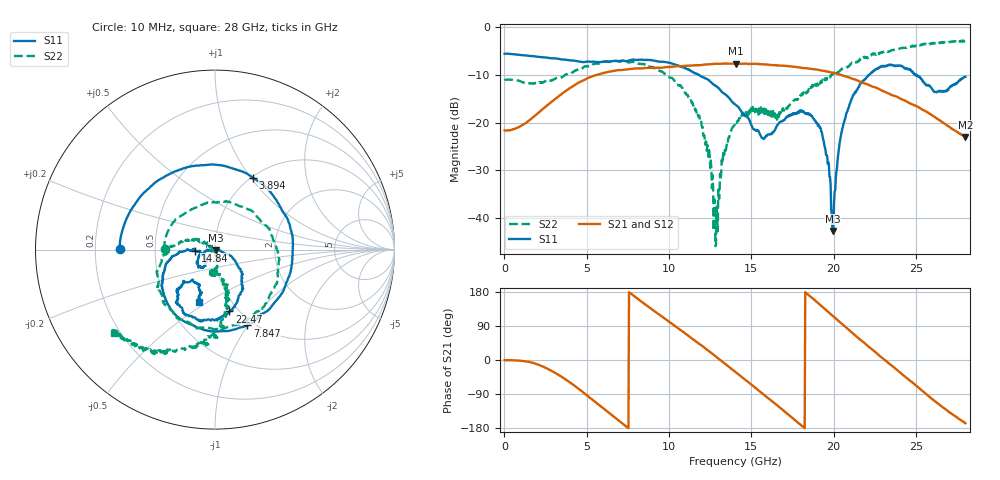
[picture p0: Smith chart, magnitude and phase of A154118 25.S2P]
!  2-Port S-parameters saved by WinCal
! VAR MeasName=S-Parameters (CALIBRATED_DATA) read from VNA (N5230A)
! VAR MeasDate=2015-9-10 14:36:17
! VAR NAME=A154118 25
! VAR FILENAME=A154118 25.S2P
! VAR DATE=2015-9-10 14:36:17
! VAR PHYS_PORTS=1,2
# Hz S DB R 50
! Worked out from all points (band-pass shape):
!   801 points, 10 MHz to 28 GHz, reference 50 ohm
!   highest |S21| = -7.57 dB at 14.07 GHz (marker M1); lowest = -23.0 dB at 28 GHz (marker M2)
!   |S21| within 3 dB of the highest: 5.095 GHz to 20.97 GHz (15.88 GHz wide, 122 % of centre)
!   lowest |S11| = -42.7 dB at 19.95 GHz (marker M3), VSWR 1.01, Z = 50.6 - j0.347 ohm
!   |S11| at or under -10 dB: 11.84 GHz to 22.14 GHz (10.3 GHz wide, 60.6 % of centre); 24.97935 GHz to 25.0482 GHz (68.84 MHz wide, 0.275 % of centre); 25.07 GHz to end of sweep
!   |S22| runs from -45.9 to -2.7 dB; largest |S21 - S12| = 0.0078
!   S11 on the Smith chart (normalised r, x): 10 MHz: 0.31, +0.00; 3.894 GHz: 1.01, +1.02; 7.847 GHz: 0.93, -0.99; 14.84 GHz: 0.80, -0.01; 22.47 GHz: 0.91, -0.71; 28 GHz: 0.71, -0.46
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1e7  -5.53 179.6  -21.62 -0.2  -21.64 0.1  -11.15 179.9
2.10925e9  -6.18 120.3  -17.80 -13.3  -17.80 -13.0  -11.46 96.2
3.893612e9  -6.87 62.3  -12.93 -56.5  -12.89 -56.5  -9.76 16.3
4.698325e9  -7.25 33.6  -11.28 -82.5  -11.26 -82.8  -8.61 -19.1
7.8472e9  -6.76 -66.9  -8.65 169.8  -8.63 169.8  -7.18 -119.2
9.351662e9  -7.15 -106.1  -8.48 121.2  -8.41 121.1  -9.05 -155.4
1.187076e10  -10.12 -155.8  -7.91 41.4  -7.84 40.8  -19.35 151.2
1.243056e10  -11.10 -165.1  -7.73 23.3  -7.66 22.5  -25.74 135.0
1.281542e10  -12.26 -170.3  -7.62 10.2  -7.56 9.5  -45.94 -44.5
1.334024e10  -13.85 -175.7  -7.58 -7.8  -7.56 -8.4  -26.83 -67.8
1.4005e10  -16.16 -179.9  -7.60 -30.6  -7.58 -31.1  -20.36 -84.3
1.407498e10  -16.33 179.8  -7.57 -33.1  -7.53 -33.5  -19.86 -82.1
1.48447e10  -19.25 -176.0  -7.67 -59.5  -7.63 -60.3  -17.98 -96.9
1.648911e10  -21.04 -125.4  -7.96 -117.2  -7.90 -117.8  -18.12 -92.4
1.869332e10  -18.63 -146.7  -8.73 163.6  -8.76 163.0  -12.08 -74.3
1.935809e10  -23.47 -163.8  -9.09 138.8  -9.12 138.1  -11.28 -75.8
1.995288e10  -42.74 -28.0  -9.53 116.2  -9.54 115.6  -9.79 -77.1
2.07226e10  -18.81 -27.1  -10.29 86.9  -10.31 86.5  -8.46 -81.2
2.247198e10  -9.03 -76.8  -12.53 23.1  -12.55 22.6  -5.64 -95.1
2.334666e10  -7.89 -99.7  -13.85 -8.9  -13.83 -9.5  -5.09 -104.3
2.618065e10  -13.54 -126.8  -18.94 -109.9  -18.92 -109.6  -3.25 -126.4
2.8e10  -10.34 -107.4  -22.98 -166.9  -23.03 -166.6  -2.72 -140.6
